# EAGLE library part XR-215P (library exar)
Monolithic PHASE-LOCKED LOOP
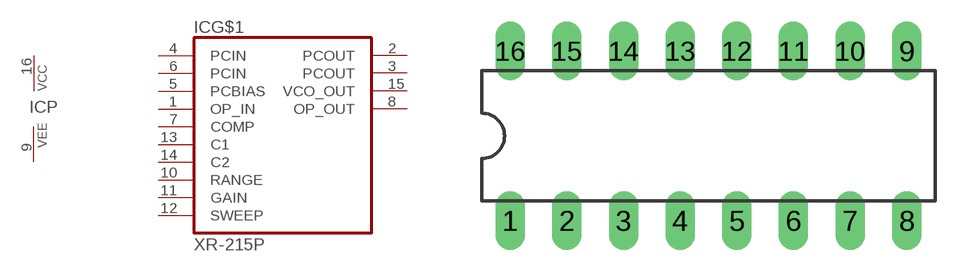
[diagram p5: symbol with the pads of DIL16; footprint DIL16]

Designator prefix IC; gates G$1=XR-215 P=PWR+/-

## XR-215P (OC_FARNELL: unknown; OC_NEWARK: unknown)  [DIL16]
1  G$1:OP_IN  in
2  G$1:PCOUT  out
3  G$1:PCOUT  out
4  G$1:PCIN  in
5  G$1:PCBIAS  in
6  G$1:PCIN  in
7  G$1:COMP  in
8  G$1:OP_OUT  out
9  P:VEE  pwr
10  G$1:RANGE  in
11  G$1:GAIN  in
12  G$1:SWEEP  in
13  G$1:C1  in
14  G$1:C2  in
15  G$1:VCO_OUT  out
16  P:VCC  pwr

## Footprint DIL16 (pad centres in mm)
Dual In Line Package
drill 0.813 long: 1 -8.89,-3.81; 2 -6.35,-3.81; 3 -3.81,-3.81; 4 -1.27,-3.81; 5 1.27,-3.81; 6 3.81,-3.81; 7 6.35,-3.81; 8 8.89,-3.81; 9 8.89,3.81; 10 6.35,3.81; 11 3.81,3.81; 12 1.27,3.81; 13 -1.27,3.81; 14 -3.81,3.81; 15 -6.35,3.81; 16 -8.89,3.81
